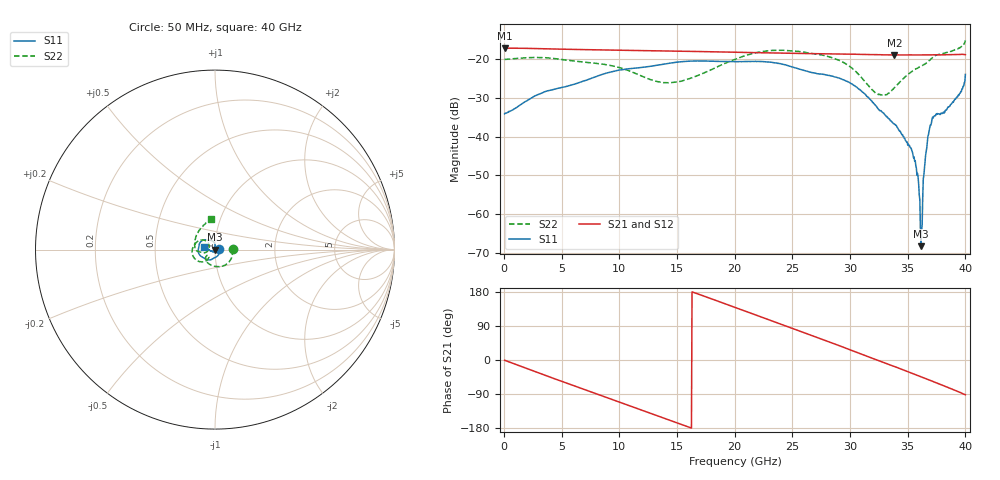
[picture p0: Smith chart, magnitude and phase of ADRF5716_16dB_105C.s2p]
! Device: ADRF5716
! Description: 30GHz 2-Bit Digital Attenuator
! Frequency: 100 MHz – 30 GHz
! Ports:
! ATTIN  = Port 1
! ATTOUT = Port 2
! State: 16 dB Attenuation selected
! Supply Voltage:
! VDD  =  +3.30 Volts
! VSS  =  -3.30 Volts
! Control Voltages:
! D5 = 3.3V, D6 = 0V
! Temperature = +105 C
! Data: Data was collected using a calibrated network analyzer.
!  The reference plane is the package pins of ADRF5716 switch.
! Note: Analog Devices supplies this data as a sample of measured data for this product.
!  Your particular data for this product may vary.
!  Analog Devices reserves the right to change this data at anytime
# HZ S DB R 50
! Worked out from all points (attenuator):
!   800 points, 50 MHz to 40 GHz, reference 50 ohm
!   highest |S21| = -17.26 dB at 100 MHz (marker M1); lowest = -19.0 dB at 33.85 GHz (marker M2)
!   lowest |S11| = -68.2 dB at 36.15 GHz (marker M3), VSWR 1.00, Z = 50 - j0.0217 ohm
!   |S11| at or under -10 dB: start of sweep to end of sweep
!   |S22| runs from -29.4 to -15.3 dB; largest |S21 - S12| = 0
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5e7  -34.17 4.3  -17.26 -0.6  -17.26 -0.6  -20.18 0.7
1e8  -33.97 0.2  -17.26 -1.2  -17.26 -1.2  -20.14 -0.9
6.75e9  -25.87 -100.8  -17.63 -75.5  -17.63 -75.5  -20.79 -97.4
1.34e10  -21.58 -150.5  -17.96 -148.4  -17.96 -148.4  -25.94 -141.5
1.56e10  -20.70 -164.9  -18.06 -172.6  -18.06 -172.6  -25.56 -129.8
2.005e10  -20.75 169.1  -18.31 138.5  -18.31 138.5  -20.09 -136.0
2.315e10  -20.89 149.3  -18.49 104.3  -18.49 104.3  -17.88 -163.2
2.67e10  -23.54 128.4  -18.68 64.4  -18.68 64.4  -18.66 166.5
3.015e10  -26.46 103.0  -18.81 25.2  -18.81 25.2  -22.37 137.7
3.225e10  -32.12 89.4  -18.94 0.9  -18.94 0.9  -28.90 152.4
3.335e10  -35.41 92.7  -19.02 -11.6  -19.02 -11.6  -28.89 -177.7
3.385e10  -36.79 95.2  -19.04 -17.3  -19.04 -17.3  -27.44 -167.8
3.545e10  -44.58 97.8  -19.01 -35.9  -19.01 -35.9  -23.09 -166.0
3.575e10  -48.15 99.6  -19.02 -39.4  -19.02 -39.4  -22.55 -167.9
3.605e10  -56.30 98.0  -19.01 -42.9  -19.01 -42.9  -22.03 -169.3
3.615e10  -68.21 -146.1  -19.03 -44.1  -19.03 -44.1  -21.94 -169.9
3.63e10  -55.73 -75.1  -19.02 -45.9  -19.02 -45.9  -21.70 -170.6
3.65e10  -46.16 -97.4  -19.01 -48.3  -19.01 -48.3  -21.33 -171.5
3.665e10  -42.90 -103.6  -19.00 -50.1  -19.00 -50.1  -20.99 -172.0
3.705e10  -36.59 -125.0  -19.00 -55.0  -19.00 -55.0  -19.93 -175.7
3.935e10  -29.72 -177.6  -18.90 -83.1  -18.90 -83.1  -17.43 135.0
4e10  -24.02 167.2  -18.94 -91.8  -18.94 -91.8  -15.29 98.0
